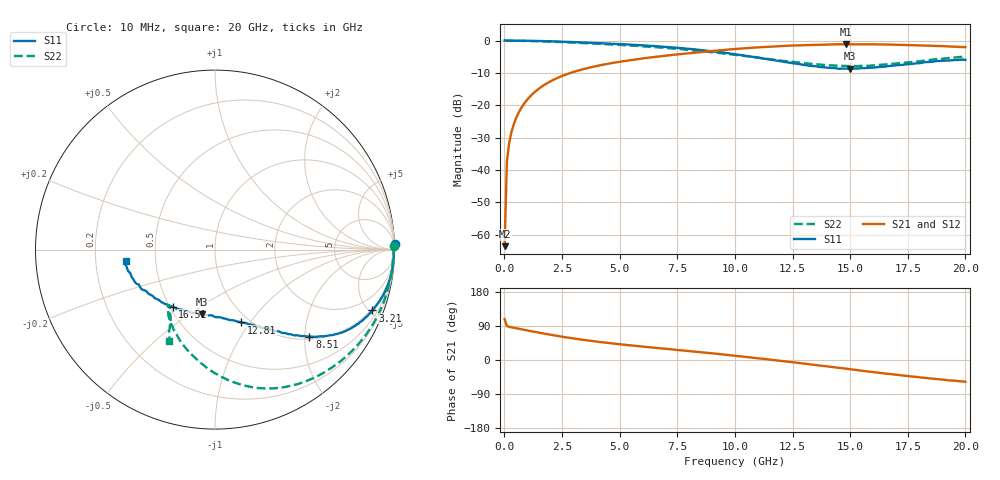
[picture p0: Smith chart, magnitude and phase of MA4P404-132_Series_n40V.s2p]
! AWR Design Environment (9226) Thu Aug 19 02:30:18 2021
! Document = 'n40V'
! nPorts: 2, nXvals: 201
# GHz S DB R 50
!Freq DBS11 AngS11 DBS21 AngS21 DBS12 AngS12 DBS22 AngS22
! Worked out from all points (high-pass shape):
!   201 points, 10 MHz to 20 GHz, reference 50 ohm
!   highest |S21| = -1.14 dB at 14.81 GHz (marker M1); lowest = -63.6 dB at 10 MHz (marker M2)
!   |S21| within 3 dB of the highest: 7.691 GHz to end of sweep
!   lowest |S11| = -8.7 dB at 15.01 GHz (marker M3), VSWR 2.15, Z = 33.8 - j28 ohm
!   |S11| at or under -10 dB: nowhere
!   |S22| runs from -7.9 to 0.0 dB; largest |S21 - S12| = 0.035
!   S11 on the Smith chart (normalised r, x): 10 MHz: -6, +63; 3.21 GHz: 0.89, -5.21; 8.51 GHz: 1.06, -2.11; 12.81 GHz: 0.91, -0.91; 16.51 GHz: 0.52, -0.39; 20 GHz: 0.33, -0.06
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0.01  0.03 1.8  -63.58 108.0  -57.12 88.2  -0.02 1.1
0.11  -0.04 -0.6  -37.27 89.5  -37.17 88.6  -0.06 -1.8
0.21  -0.04 -1.5  -31.63 87.5  -31.66 87.1  -0.06 -3.4
0.31  -0.03 -2.2  -28.26 86.2  -28.27 86.1  -0.06 -5.1
0.51  -0.03 -3.7  -23.96 83.8  -23.96 83.8  -0.08 -8.3
0.91  -0.06 -6.7  -19.00 79.0  -19.01 79.1  -0.12 -14.8
1.51  -0.14 -11.0  -14.80 72.0  -14.81 72.3  -0.22 -24.1
2.21  -0.27 -15.6  -11.85 64.4  -11.86 64.8  -0.40 -34.0
3.21  -0.53 -21.1  -9.26 55.1  -9.25 55.6  -0.71 -46.3
3.41  -0.59 -22.2  -8.86 53.3  -8.86 53.9  -0.77 -48.5
5.01  -1.10 -29.3  -6.56 41.6  -6.55 42.4  -1.35 -63.6
6.71  -1.80 -35.7  -4.92 31.3  -4.87 32.3  -2.13 -76.6
8.51  -2.91 -42.7  -3.56 20.7  -3.50 21.9  -3.24 -90.1
10.01  -4.19 -49.4  -2.62 11.2  -2.54 12.6  -4.43 -102.3
12.81  -7.30 -70.2  -1.45 -8.2  -1.40 -7.0  -6.82 -124.3
13.41  -7.90 -77.1  -1.32 -12.5  -1.27 -11.3  -7.27 -127.2
14.81  -8.67 -97.6  -1.14 -22.9  -1.14 -21.5  -7.85 -129.5
15.01  -8.74 -101.5  -1.15 -24.5  -1.13 -23.1  -7.87 -129.8
16.51  -8.06 -126.7  -1.22 -35.6  -1.23 -33.4  -7.40 -126.2
16.71  -7.87 -129.2  -1.26 -37.0  -1.24 -34.9  -7.28 -125.3
18.91  -6.28 -160.4  -1.70 -51.3  -1.69 -49.7  -5.65 -119.3
20  -5.98 -172.6  -2.04 -57.5  -2.06 -55.9  -4.93 -116.6
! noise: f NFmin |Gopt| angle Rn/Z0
0.01  0  1  0  2e-20
2.21  0  1  0  2e-20
4.41  0  1  0  2e-20
6.61  0  1  0  2e-20
8.81  0  1  0  2e-20
11.11  0  1  0  2e-20
13.31  0  1  0  2e-20
15.51  0  1  0  2e-20
17.71  0  1  0  2e-20
20  0  1  0  2e-20
